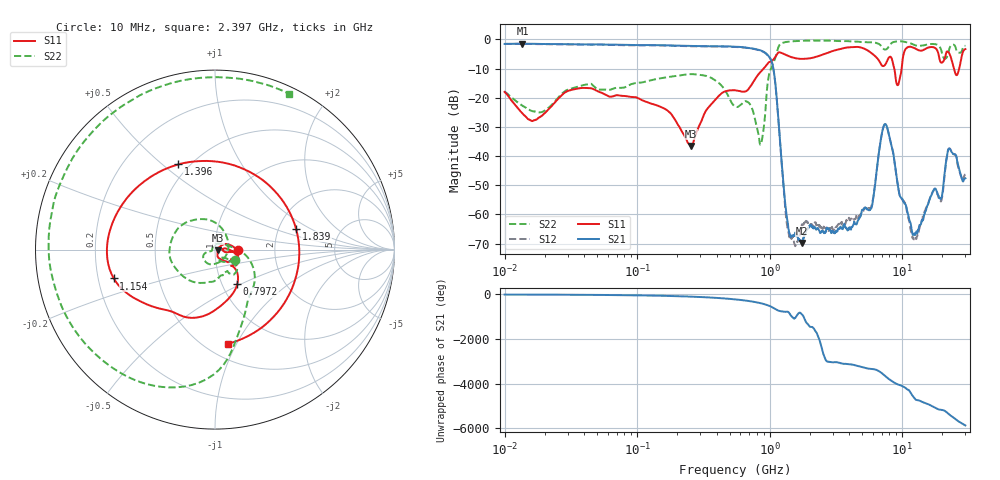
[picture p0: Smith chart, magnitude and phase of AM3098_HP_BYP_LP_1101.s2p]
!Agilent Technologies,E8364B,MY43040894,A.07.50.67
!Agilent E8364B: A.07.50.67
!Date: Wednesday, June 17, 2020 09:21:48
!Correction: S11(Full 2 Port(1,2))
!S21(Full 2 Port(1,2))
!S12(Full 2 Port(1,2))
!S22(Full 2 Port(1,2))
!S2P File: Measurements: S11, S21, S12, S22:Log Frequency Sweep
# Hz S  dB  R 50
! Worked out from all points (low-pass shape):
!   1601 points, 10 MHz to 30 GHz, reference 50 ohm
!   highest |S21| = -1.41 dB at 13.64 MHz (marker M1); lowest = -69.8 dB at 1.758 GHz (marker M2)
!   |S21| within 3 dB of the highest: start of sweep to 916.3 MHz
!   lowest |S11| = -36.5 dB at 254.7 MHz (marker M3), VSWR 1.03, Z = 51.4 - j0.448 ohm
!   |S11| at or under -10 dB: start of sweep to 900 MHz; 8.723 GHz to 9.912 GHz (1.189 GHz wide, 12.8 % of centre); 24.61 GHz to 26.93 GHz (2.314 GHz wide, 8.98 % of centre)
!   |S22| runs from -36.1 to -0.3 dB; largest |S21 - S12| = 0.014
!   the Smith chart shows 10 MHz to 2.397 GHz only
!   S11 on the Smith chart (normalised r, x): 10 MHz: 1.29, -0.00; 797.2 MHz: 1.18, -0.48; 1.154 GHz: 0.27, -0.13; 1.396 GHz: 0.44, +0.57; 1.839 GHz: 2.48, +0.74; 2.397 GHz: 0.64, -0.93
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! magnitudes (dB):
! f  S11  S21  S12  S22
! 10 MHz  -18.0  -1.5  -1.5  -17.9
! 13.64 MHz  -25.3  -1.4  -1.5  -22.8
! 38.04 MHz  -16.6  -1.7  -1.7  -15.8
! 144.7 MHz  -22.8  -2.0  -2.0  -13.4
! 254.7 MHz  -36.5  -2.2  -2.3  -11.9
! 547.7 MHz  -17.4  -2.5  -2.6  -23.0
! 797.2 MHz  -12.8  -3.4  -3.5  -30.0
! 876.7 MHz  -10.6  -3.9  -4.1  -34.3
! 1.029 GHz  -7.5  -7.2  -7.3  -9.8
! 1.154 GHz  -4.6  -25.2  -25.4  -3.1
! 1.396 GHz  -5.7  -65.5  -66.7  -0.7
! 1.758 GHz  -6.7  -69.8  -63.4  -0.5
! 1.839 GHz  -6.6  -67.0  -62.7  -0.4
! 2.084 GHz  -6.3  -64.0  -63.5  -0.4
! 2.397 GHz  -5.5  -66.3  -64.2  -0.3
! 5.725 GHz  -4.3  -58.5  -57.9  -1.0
! 7.135 GHz  -9.1  -30.8  -30.9  -2.9
! 7.926 GHz  -6.2  -32.4  -32.5  -2.4
! 9.302 GHz  -15.6  -50.4  -50.5  -0.7
! 12.31 GHz  -2.9  -66.6  -68.4  -1.8
! 22.67 GHz  -4.8  -37.4  -37.4  -3.3
! 30 GHz  -3.3  -47.6  -46.3  -2.2
